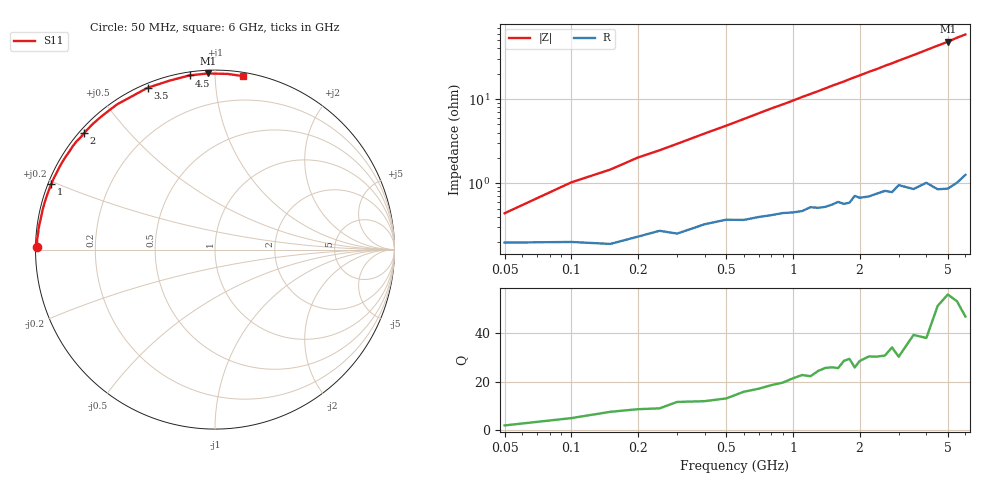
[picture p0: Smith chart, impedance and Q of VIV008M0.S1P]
! Infineon Technologies  Discrete & RF Semiconductors
! BB 804
! Si Tuning Diode in SOT23
! VR =
! S-Parameters:  July  1999
# GHz  S  MA  R  50
!  f  S11
! GHz  MAG  ANG
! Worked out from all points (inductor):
!   34 points, 50 MHz to 6 GHz, reference 50 ohm
!   read as one part to ground: L = 1.6 nH near 100 MHz
!   highest Q = 52.9 at 5 GHz (marker M1), where L = 1.53 nH
!   S11 on the Smith chart (normalised r, x): 50 MHz: 0.00, +0.01; 1 GHz: 0.01, +0.19; 2 GHz: 0.01, +0.38; 3.5 GHz: 0.02, +0.67; 4.5 GHz: 0.02, +0.86; 6 GHz: 0.03, +1.17
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0.05  0.9922 179.1
0.1  0.992 177.7
0.15  0.9925 176.7
0.2  0.9908 175.4
0.25  0.9892 174.4
0.3  0.99 173.3
0.6  0.9857 166.8
0.8  0.9838 162.4
1  0.9828 158.3
1.1  0.9823 156.1
1.3  0.981 152.1
1.5  0.9797 147.9
1.6  0.9784 146.0
1.7  0.9797 144.1
1.8  0.9792 142.0
1.9  0.9754 140.0
2  0.9768 138.2
2.2  0.9767 134.3
2.4  0.9753 130.9
2.6  0.9743 127.1
2.8  0.9759 123.9
3  0.9718 120.4
3.5  0.9767 112.6
4  0.9748 105.1
4.5  0.9808 98.3
5  0.9822 92.3
5.5  0.9813 85.9
6  0.9791 80.9
